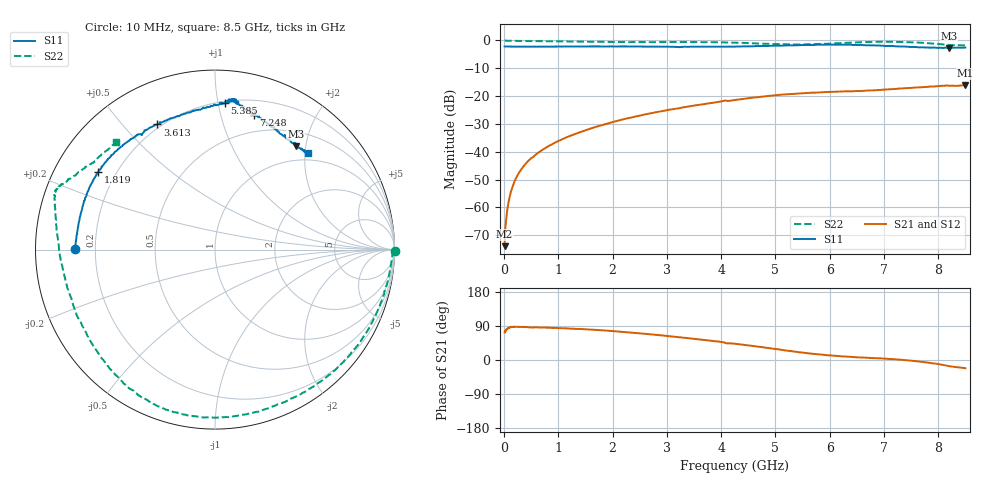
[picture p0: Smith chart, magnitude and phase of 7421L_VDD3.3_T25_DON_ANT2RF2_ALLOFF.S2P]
!Agilent Technologies,E5071C,MY46417908,A.11.23
!Date: Thu Feb 25 16:17:37 2021
!Data & Calibration Information:
!Freq	S11:SOLT2(ON)	S21:SOLT2(ON)	S12:SOLT2(ON)	S22:SOLT2(ON)
!PortZ  Port1:50+j0  Port2:50+j0
!Above PortZ is port z conversion or system Z0 setting when saving the data.
!When reading, reference impedance value at option line is always used.
# Hz S dB R 50
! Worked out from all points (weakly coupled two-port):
!   1601 points, 10 MHz to 8.5 GHz, reference 50 ohm
!   highest |S21| = -16.14 dB at 8.5 GHz (marker M1); lowest = -73.9 dB at 10 MHz (marker M2)
!   lowest |S11| = -2.7 dB at 8.198 GHz (marker M3), VSWR 6.43, Z = 36.8 + j90.9 ohm
!   |S11| at or under -10 dB: nowhere
!   |S22| runs from -1.8 to 0.0 dB; largest |S21 - S12| = 0.0027
!   S11 on the Smith chart (normalised r, x): 10 MHz: 0.12, +0.00; 1.819 GHz: 0.13, +0.30; 3.613 GHz: 0.18, +0.62; 5.385 GHz: 0.21, +1.05; 7.248 GHz: 0.33, +1.28; 8.5 GHz: 0.85, +2.06
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1e7  -2.14 179.7  -73.93 72.6  -74.29 82.6  0.00 -0.4
6.836875e7  -2.18 178.5  -59.72 83.2  -59.57 84.1  -0.10 -2.1
1.214312e8  -2.19 177.3  -54.68 87.4  -54.66 86.9  -0.12 -3.5
2.116375e8  -2.21 175.4  -49.83 87.6  -49.85 87.4  -0.15 -5.8
3.336812e8  -2.22 172.9  -45.90 87.4  -45.83 87.4  -0.18 -9.0
4.822562e8  -2.23 169.8  -42.63 86.1  -42.62 86.2  -0.23 -12.8
7.741e8  -2.22 164.4  -38.51 85.4  -38.51 85.6  -0.28 -20.2
1.426769e9  -2.15 152.9  -32.77 81.6  -32.77 81.7  -0.42 -38.1
1.819431e9  -2.14 146.3  -30.30 78.2  -30.30 78.1  -0.51 -49.4
2.339444e9  -2.14 137.8  -27.69 72.3  -27.69 72.3  -0.59 -65.3
2.843538e9  -2.23 129.1  -25.64 65.7  -25.64 65.7  -0.60 -80.5
3.612944e9  -2.29 114.8  -23.06 54.1  -23.06 54.1  -0.59 -102.1
4.255e9  -2.19 101.8  -21.40 42.9  -21.41 42.8  -0.79 -118.8
4.843994e9  -1.96 91.7  -20.00 32.2  -19.98 32.0  -1.21 -137.5
5.385231e9  -1.71 86.1  -19.09 21.5  -19.06 21.7  -1.44 -160.2
5.671769e9  -1.65 84.5  -18.77 16.7  -18.71 16.9  -1.37 -172.4
6.393419e9  -1.56 83.3  -18.28 8.2  -18.34 8.7  -0.77 166.5
7.088538e9  -1.97 75.9  -17.55 2.8  -17.60 2.4  -0.45 159.7
7.247725e9  -2.14 73.9  -17.33 1.4  -17.34 1.4  -0.51 158.8
7.751819e9  -2.51 62.9  -16.72 -5.8  -16.75 -5.8  -0.88 154.2
8.197544e9  -2.72 51.9  -16.28 -16.3  -16.33 -16.5  -1.64 143.5
8.5e9  -2.54 46.0  -16.14 -21.9  -16.23 -22.4  -1.79 132.7
